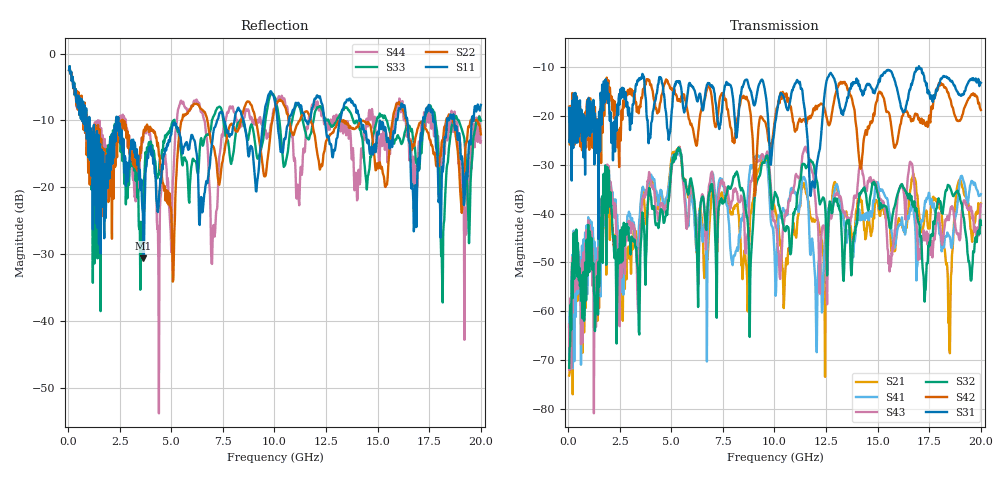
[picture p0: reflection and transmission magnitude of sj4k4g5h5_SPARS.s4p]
! FILE: E:\users\goganessyan\GBX_Backplane\FR408_backplane\1m_OUTBOUND_NEXT\sj4k4g5h5_SPARS.s4p
# MHZ S RI R 50.00
! FREQ  S11  S12  S13  S14
!  S21  S22  S23  S24
!  S31  S32  S33  S34
!  S41  S42  S43  S44
!  REAL  IMAG  REAL  IMAG  REAL  IMAG  REAL  IMAG
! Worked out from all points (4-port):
!   799 points, 50 MHz to 20 GHz, reference 50 ohm
!   strongest paths, dB at 50 MHz, 5.025 GHz, 10.03 GHz, 15.03 GHz, 20 GHz:
!     S31: -18.4, -18.8, -21.6, -13.5, -13.3
!     S42: -18.1, -14.7, -20.6, -15.5, -18.8
!     S32: -71.6, -29.8, -35.6, -36.8, -42.3
!     S43: -62.8, -30.6, -41.5, -35.9, -38.1
!     S41: -63.2, -29.7, -51.2, -33.9, -36.0
!     S21: -73.2, -28.5, -39.1, -38.3, -37.9
!   lowest |S11| = -30.7 dB at 3.65 GHz (marker M1), VSWR 1.06, Z = 50.2 + j2.93 ohm
!   |S11| at or under -10 dB: 1.027 GHz to 2.333 GHz (1.306 GHz wide, 77.7 % of centre); 2.434 GHz to 7.223 GHz (4.789 GHz wide, 99.2 % of centre); 14.18 GHz to 15.89 GHz (1.708 GHz wide, 11.4 % of centre)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
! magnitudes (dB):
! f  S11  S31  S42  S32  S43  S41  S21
! 50 MHz  -2.5  -18.4  -18.1  -71.6  -62.8  -63.2  -73.2
! 3.65 GHz  -30.7  -12.0  -14.5  -41.6  -36.6  -35.0  -35.5
! 10.28 GHz  -14.0  -15.8  -16.3  -39.4  -53.4  -40.2  -46.6
! 11.43 GHz  -9.1  -17.5  -20.7  -29.8  -27.0  -32.5  -33.8
! 12.03 GHz  -6.5  -30.9  -18.4  -32.9  -39.9  -66.1  -41.3
! 18.48 GHz  -9.8  -12.5  -16.2  -34.3  -40.5  -44.7  -67.8
! 20 GHz  -7.7  -13.3  -18.8  -42.3  -38.1  -36.0  -37.9
